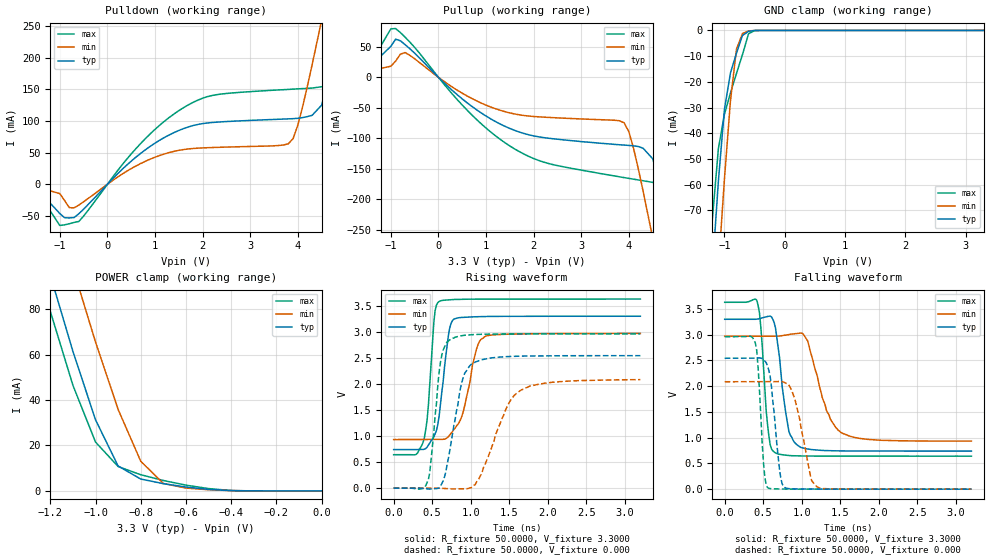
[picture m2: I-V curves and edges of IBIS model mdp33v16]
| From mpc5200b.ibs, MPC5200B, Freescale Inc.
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|   Model mdp33v16
[Model]   mdp33v16
Model_type   I/O
Polarity   Non-Inverting
Enable   Active-High
Vinl =   0.8000V
Vinh =   2.0000V
Vmeas =   1.5000V
C_comp   2.1096pF   1.4802pF   2.7108pF
[Temperature Range]   27.0000   0.1250k   -40.0000
[Voltage Range]   3.3000V   2.9700V   3.6300V
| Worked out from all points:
|   slope of the pulldown table from 0 to 0.495 V, typ, clamps not added: 13.7 ohm
|   slope of the pullup table from 0 to 0.495 V, typ, clamps not added: 14.1 ohm
|   GND clamp passes 1 mA (typ) near -0.64 V on its own axis
|   POWER clamp passes 1 mA (typ) near -0.53 V on its own axis
|   rising waveform, R_fixture 50.0000, V_fixture 3.3000: 20-80 % time 122ps typ, 182ps min, 86.6ps max; typ from 0.74 V to 3.3 V
|   rising waveform, R_fixture 50.0000, V_fixture 0.000: 20-80 % time 184ps typ, 336ps min, 115ps max; typ from 0 V to 2.54 V
|   falling waveform, R_fixture 50.0000, V_fixture 3.3000: 20-80 % time 127ps typ, 246ps min, 82.5ps max; typ from 3.3 V to 0.74 V
|   falling waveform, R_fixture 50.0000, V_fixture 0.000: 20-80 % time 99.6ps typ, 169ps min, 66.5ps max; typ from 2.54 V to 0 V
[Pulldown]
| voltage   I(typ)   I(min)   I(max)
-3.3V     -1.992mA   -1.655mA   -1.685mA
-1.5V     -5.553mA   -4.034mA   -7.836mA
-1V       -46.21mA   -14.74mA   -65.11mA
-600mV    -46.59mA   -32.86mA   -58.79mA
700mV     48.9mA     32.81mA    64.5mA
1.7V      90.52mA    55.82mA    125.4mA
3.8V      103.3mA    63.92mA    149.8mA
4V        104.2mA    93.46mA    150.7mA
4.5V      125mA      259.4mA    154mA
4.9V      254.4mA    404.9mA    165.8mA
5.3V      402.5mA    553.3mA    270.9mA
6.6V      905.4mA    1.045A     773.7mA
[Pullup]
| voltage   I(typ)   I(min)   I(max)
-3.3V     5.492mA    7.76mA     5.435mA
-1.5V     12.97mA    9.901mA    13.14mA
-900mV    62.58mA    26.52mA    80.05mA
-700mV    53.62mA    40.6mA     65.83mA
700mV     -47.64mA   -34.74mA   -61.65mA
1.7V      -89.86mA   -61.59mA   -122mA
3.9V      -111.2mA   -74.69mA   -164.6mA
4.1V      -112.5mA   -117.3mA   -167.2mA
4.5V      -133.7mA   -263.9mA   -172.4mA
4.9V      -257.7mA   -423.2mA   -197.1mA
5.3V      -416.6mA   -585.8mA   -269.8mA
6.6V      -951.6mA   -1.122A    -796.3mA
[GND_clamp]
| voltage   I(typ)   I(min)   I(max)
-3.3V     -948.1mA   -982.8mA   -929.6mA
-1.3V     -130.7mA   -168mA     -108.8mA
-1.2V     -93.35mA   -129.8mA   -73.5mA
-1.1V     -58.65mA   -92.83mA   -45.99mA
-1V       -30.69mA   -57.94mA   -32.68mA
-900mV    -16.54mA   -27.44mA   -24.36mA
-800mV    -8.854mA   -7.262mA   -16.75mA
-700mV    -1.936mA   -1.183mA   -9.358mA
-600mV    -366uA     -212.8uA   -1.293mA
-500mV    -39.22uA   -34.56uA   -92.73uA
3.3V      541.3pA    33.88uA    287.7pA
[POWER_clamp]
| voltage   I(typ)   I(min)   I(max)
-3.3V     897.6mA    912.2mA    893.7mA
-1.3V     130.2mA    167.4mA    114.6mA
-1.2V     95.06mA    132.3mA    79.13mA
-1.1V     61.46mA    98.2mA     46.53mA
-1V       31.32mA    65.57mA    21.52mA
-900mV    10.96mA    35.88mA    10.75mA
-800mV    5.231mA    13.06mA    7.129mA
-700mV    3.197mA    3.28mA     4.595mA
-600mV    1.712mA    1.263mA    2.547mA
-500mV    672.1uA    514.1uA    1.035mA
-400mV    127.3uA    134.7uA    183.8uA
0V        541.3pA    4.807nA    325.5pA
[Ramp]
| variable   typ   min   max
dV/dt_r   1.5215/0.1828n   1.1497/0.2913n   1.7764/0.1140n
dV/dt_f   1.5354/0.1253n   1.1819/0.2303n   1.7931/77.2955p
R_load = 50.0000
[Rising Waveform]
R_fixture = 50.0000
V_fixture = 3.3000
V_fixture_min = 2.9700
V_fixture_max = 3.6300
| time   V(typ)   V(min)   V(max)
0s        739.8mV    932.5mV    641.4mV
381.6ps   741.4mV    932.7mV    878.3mV
433.7ps   787.2mV    932.7mV    1.306V
537.8ps   1.045V     932mV      3.412V
589.8ps   1.382V     931.5mV    3.582V
711.2ps   2.942V     991.2mV    3.615V
780.6ps   3.244V     1.122V     3.621V
1.093ns   3.292V     2.749V     3.629V
1.197ns   3.295V     2.92V      3.629V
3.2ns     3.3V       2.97V      3.63V
[Rising Waveform]
R_fixture = 50.0000
V_fixture = 0.000
| time   V(typ)   V(min)   V(max)
0s        31.3nV     102.6nV    74.89nV
381.6ps   -6.846mV   86.58uV    -5.192mV
451ps     -17.44mV   218.6uV    168.1mV
607.1ps   32.79mV    -2.465mV   2.413V
745.9ps   879.2mV    -15.48mV   2.866V
902ps     2.12V      -14.94mV   2.931V
1.058ns   2.421V     69.17mV    2.95V
1.457ns   2.524V     1.522V     2.96V
1.648ns   2.534V     1.879V     2.961V
3.2ns     2.543V     2.083V     2.961V
[Falling Waveform]
R_fixture = 50.0000
V_fixture = 3.3000
V_fixture_min = 2.9700
V_fixture_max = 3.6300
| time   V(typ)   V(min)   V(max)
0s        3.3V       2.97V      3.63V
416.3ps   3.303V     2.97V      3.668V
468.4ps   3.322V     2.97V      3.153V
572.4ps   3.358V     2.97V      1.042V
659.2ps   3.128V     2.969V     702.5mV
832.7ps   1.121V     3.003V     653.8mV
971.4ps   825.5mV    3.029V     645.6mV
1.318ns   749.3mV    1.538V     641.7mV
1.509ns   743.1mV    1.099V     641.5mV
3.2ns     739.8mV    932.8mV    641.4mV
[Falling Waveform]
R_fixture = 50.0000
V_fixture = 0.000
| time   V(typ)   V(min)   V(max)
0s        2.543V     2.087V     2.961V
399ps     2.545V     2.087V     2.831V
433.7ps   2.55V      2.087V     2.354V
503.1ps   2.519V     2.086V     510.6mV
555.1ps   2.394V     2.087V     31.23mV
711.2ps   384.8mV    2.093V     3.56mV
780.6ps   31.21mV    2.067V     2.161mV
902ps     5.507mV    1.783V     930.5uV
1.197ns   1.251mV    47.92mV    94.99uV
3.2ns     8.414uV    8.427uV    2.175uV
